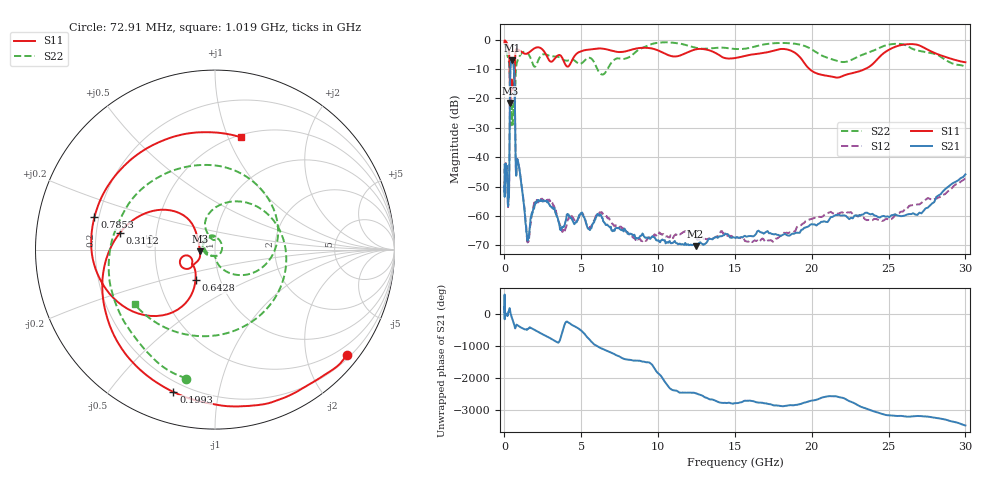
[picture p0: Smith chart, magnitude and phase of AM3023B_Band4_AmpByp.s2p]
# Hz S DB R 50.0
!freq dBS11 angS11 dBS21 angS21 dBS12 angS12 dBS22 angS22
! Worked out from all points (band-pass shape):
!   1601 points, 10 MHz to 30 GHz, reference 50 ohm
!   highest |S21| = -7.02 dB at 483.3 MHz (marker M1); lowest = -70.3 dB at 12.43 GHz (marker M2)
!   |S21| within 3 dB of the highest: 384.7 MHz to 617.5 MHz (232.8 MHz wide, 46.5 % of centre)
!   lowest |S11| = -21.5 dB at 372.6 MHz (marker M3), VSWR 1.18, Z = 42.3 - j0.766 ohm
!   |S11| at or under -10 dB: 334.7 MHz to 668.6 MHz (333.9 MHz wide, 66.6 % of centre); 19.86 GHz to 23.47 GHz (3.607 GHz wide, 16.7 % of centre)
!   |S22| runs from -29.2 to -0.9 dB; largest |S21 - S12| = 0.017
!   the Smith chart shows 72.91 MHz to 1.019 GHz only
!   S11 on the Smith chart (normalised r, x): 72.91 MHz: 0.28, -2.84; 199.3 MHz: 0.15, -0.74; 311.2 MHz: 0.30, +0.08; 642.8 MHz: 0.76, -0.27; 785.3 MHz: 0.18, +0.13; 1.019 GHz: 0.53, +1.12
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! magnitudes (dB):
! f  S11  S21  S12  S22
! 10 MHz  -0.4  -42.6  -45.7  -1.0
! 17.17 MHz  -1.2  -53.2  -48.8  -1.6
! 38.04 MHz  -0.3  -46.1  -46.2  -1.6
! 72.91 MHz  -0.5  -42.4  -42.9  -2.7
! 144.7 MHz  -1.0  -44.6  -43.5  -4.5
! 199.3 MHz  -1.7  -50.0  -50.8  -5.5
! 242.3 MHz  -2.4  -56.4  -56.5  -6.3
! 311.2 MHz  -5.4  -47.7  -47.1  -8.5
! 372.6 MHz  -21.5  -12.1  -12.1  -24.7
! 483.3 MHz  -13.6  -7.0  -7.0  -23.2
! 547.7 MHz  -17.1  -7.3  -7.3  -28.1
! 642.8 MHz  -14.0  -12.8  -12.7  -25.3
! 735.8 MHz  -3.6  -43.0  -42.7  -11.1
! 785.3 MHz  -3.2  -43.4  -43.7  -8.3
! 1.019 GHz  -3.9  -45.7  -45.7  -5.3
! 1.528 GHz  -4.6  -67.9  -68.5  -4.7
! 2.084 GHz  -2.6  -55.4  -54.7  -8.5
! 7.926 GHz  -3.9  -65.2  -65.5  -6.3
! 12.43 GHz  -3.3  -70.3  -66.9  -2.7
! 21.45 GHz  -12.7  -60.0  -59.3  -6.9
! 26.21 GHz  -1.5  -59.5  -57.5  -2.1
! 30 GHz  -7.7  -45.8  -47.2  -9.1
